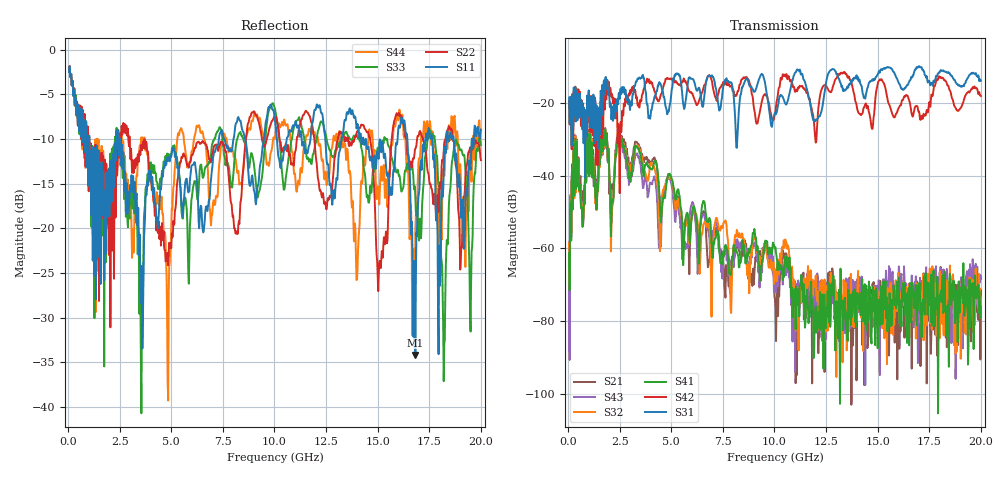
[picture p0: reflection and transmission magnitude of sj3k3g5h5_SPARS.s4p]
! FILE: E:\users\goganessyan\GBX_Backplane\FR408_backplane\1m_OUTBOUND_FEXT\sj3k3g5h5_SPARS.s4p
# MHZ S RI R 50.00
! FREQ  S11  S12  S13  S14
!  S21  S22  S23  S24
!  S31  S32  S33  S34
!  S41  S42  S43  S44
!  REAL  IMAG  REAL  IMAG  REAL  IMAG  REAL  IMAG
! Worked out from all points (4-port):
!   799 points, 50 MHz to 20 GHz, reference 50 ohm
!   strongest paths, dB at 50 MHz, 5.025 GHz, 10.03 GHz, 15.03 GHz, 20 GHz:
!     S31: -18.5, -16.1, -22.6, -11.9, -13.8
!     S42: -19.4, -13.5, -22.8, -14.1, -18.0
!     S41: -61.2, -41.1, -60.0, -80.7, -76.1
!     S32: -58.5, -41.1, -65.7, -76.7, -73.6
!     S43: -59.8, -43.1, -68.6, -83.5, -68.5
!     S21: -58.4, -41.8, -73.9, -77.6, -71.5
!   lowest |S11| = -34.2 dB at 16.82 GHz (marker M1), VSWR 1.04, Z = 48.7 - j1.42 ohm
!   |S11| at or under -10 dB: 1.027 GHz to 2.322 GHz (1.296 GHz wide, 77.4 % of centre); 2.504 GHz to 7.307 GHz (4.803 GHz wide, 97.9 % of centre); 14.43 GHz to 15.96 GHz (1.537 GHz wide, 10.1 % of centre)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
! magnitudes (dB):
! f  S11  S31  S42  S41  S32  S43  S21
! 50 MHz  -2.5  -18.5  -19.4  -61.2  -58.5  -59.8  -58.4
! 350 MHz  -5.7  -15.6  -15.4  -29.8  -29.1  -29.8  -28.8
! 2.45 GHz  -10.3  -17.3  -26.2  -29.2  -29.1  -30.3  -28.5
! 3.525 GHz  -28.4  -13.0  -19.6  -34.8  -34.1  -37.9  -33.2
! 11.1 GHz  -8.7  -10.7  -16.7  -75.3  -75.5  -72.9  -82.3
! 16.82 GHz  -34.2  -10.7  -20.9  -74.3  -72.3  -70.7  -72.6
! 20 GHz  -9.0  -13.8  -18.0  -76.1  -73.6  -68.5  -71.5
